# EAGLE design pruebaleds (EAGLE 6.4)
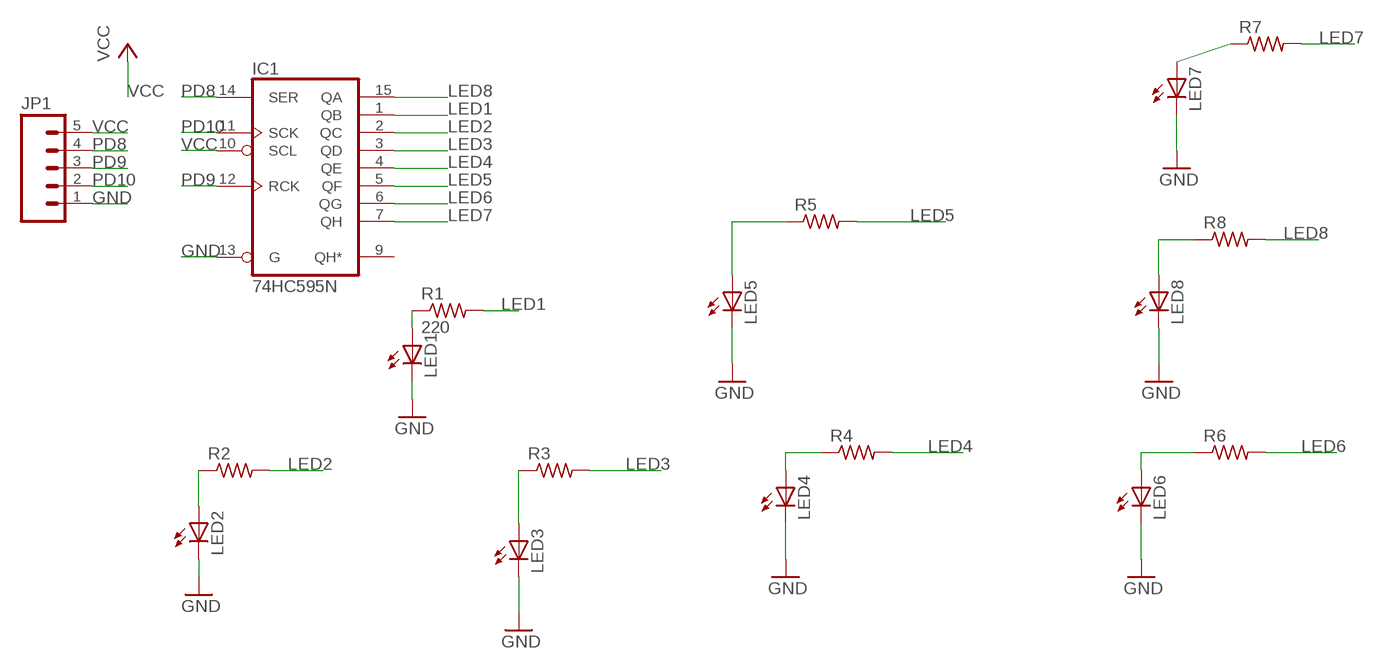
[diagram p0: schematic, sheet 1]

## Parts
IC1  74HC595N  [DIL16]
JP1  M05PTH  [1X05]
LED1  LED1206  [1206]
LED2  LED1206  [1206]
LED3  LED1206  [1206]
LED4  LED1206  [1206]
LED5  LED1206  [1206]
LED6  LED1206  [1206]
LED7  LED1206  [1206]
LED8  LED1206  [1206]
R1  220  RESISTOR1206  [1206]
R2  RESISTOR1206  [1206]
R3  RESISTOR1206  [1206]
R4  RESISTOR1206  [1206]
R5  RESISTOR1206  [1206]
R6  RESISTOR1206  [1206]
R7  RESISTOR1206  [1206]
R8  RESISTOR1206  [1206]

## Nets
GND: IC1.13(G) JP1.1 LED1.2(C) LED2.2(C) LED3.2(C) LED4.2(C) LED5.2(C) LED6.2(C) LED7.2(C) LED8.2(C)
LED1: IC1.1(QB) R1.2
LED2: IC1.2(QC) R2.2
LED3: IC1.3(QD) R3.2
LED4: IC1.4(QE) R4.2
LED5: IC1.5(QF) R5.2
LED6: IC1.6(QG) R6.2
LED7: IC1.7(QH) R7.2
LED8: IC1.15(QA) R8.2
N$1: LED2.1(A) R2.1
N$2: LED3.1(A) R3.1
N$3: LED4.1(A) R4.1
N$4: LED6.1(A) R6.1
N$5: LED8.1(A) R8.1
N$6: LED5.1(A) R5.1
N$7: LED7.1(A) R7.1
N$8: LED1.1(A) R1.1
PD8: IC1.14(SER) JP1.4
PD9: IC1.12(RCK) JP1.3
PD10: IC1.11(SCK) JP1.2
VCC: IC1.10(SCL) JP1.5
Unconnected: IC1.9(QH*)

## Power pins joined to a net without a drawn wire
GND: IC1.8(GND)
VCC: IC1.16(VCC)

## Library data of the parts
IC1 = 74xx-eu:74*595: 8-bit SHIFT REGISTER, output latch
JP1 = 01_SparkFun:M05: Header 5 Standard 5-pin 0.1" header. Use with straight break away headers (SKU : PRT-00116), right angle break away headers (PRT-00553), swiss pins (PRT-00743), machine pins (PRT-00117), and female headers (PRT-00115). Molex polarized connector foot print use with SKU : PRT-08230 with associated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
LED1-LED8 = 01_FAB_Hello:LED
R1-R8 = 01_FAB_Hello:RESISTOR

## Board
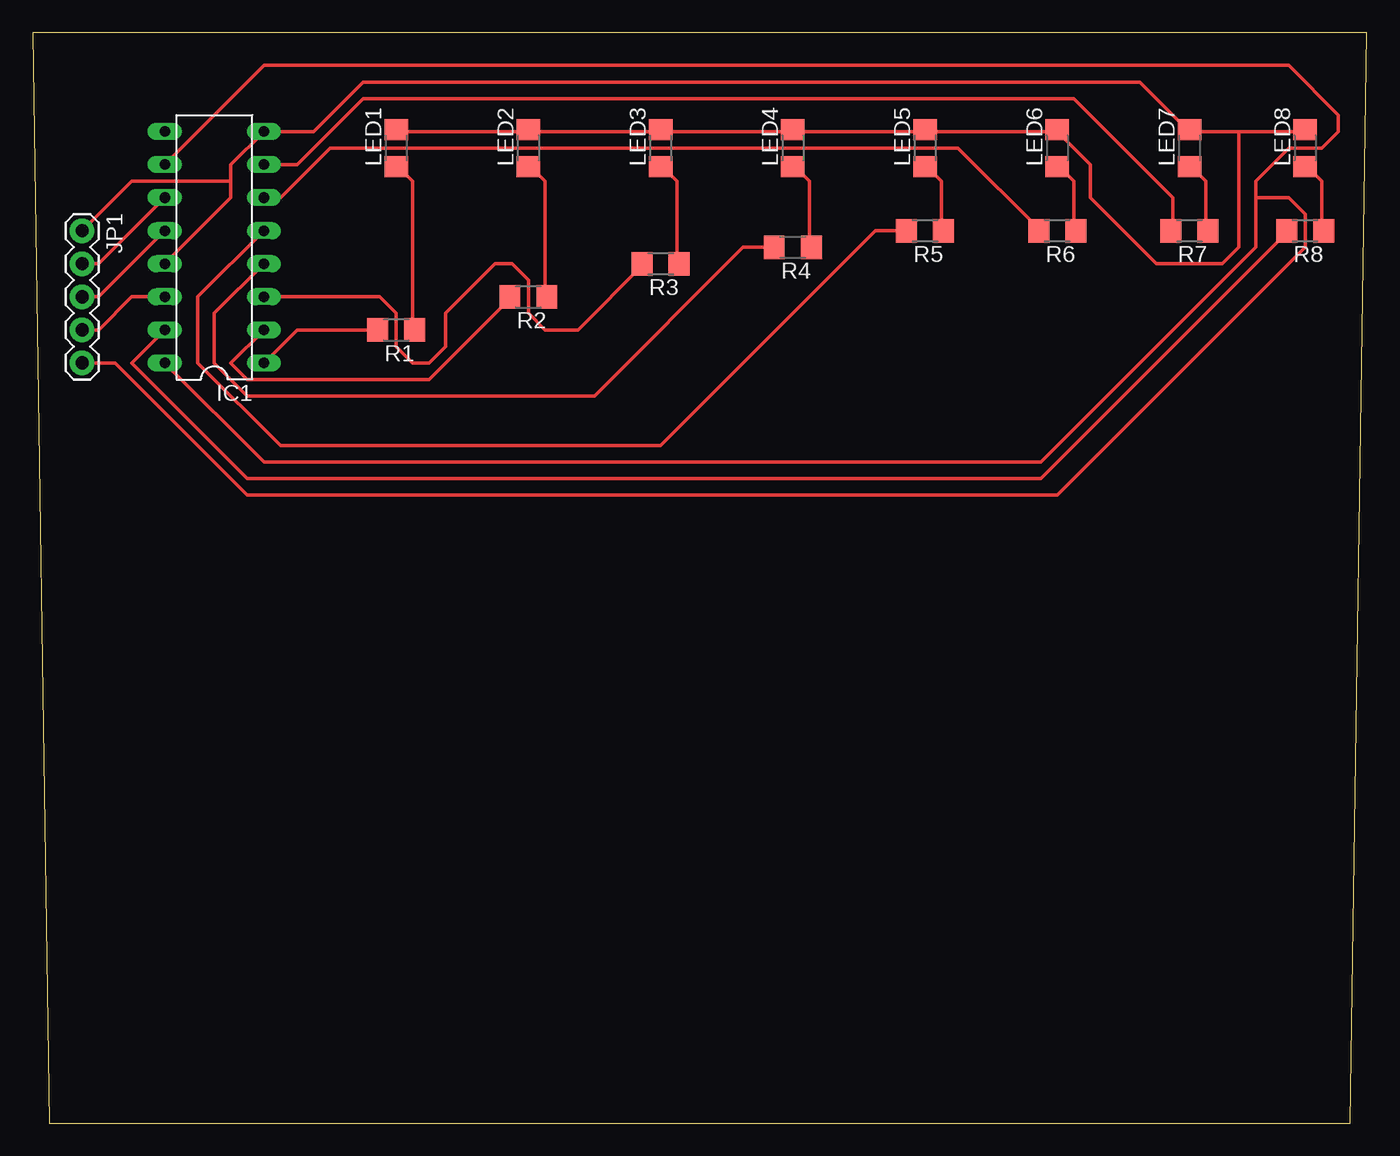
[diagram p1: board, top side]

Size 102.54 x 83.81 mm. Coordinates in mm from the lower left corner, seen from the top.
Outline: 1.27,0 101.27,0 102.54,83.81 0,83.81 1.27,0
Copper layers (1*16): Top 0.035mm / dielectric 1.5mm / Bottom 0.035mm
Design rules "default *": minimum track width 10mil, minimum drill 24mil, track to track 16mil, track to pad 16mil, pad to pad 16mil, via to via 16mil, smd to smd 0mil, copper to edge 40mil, drill to drill 8mil, minimum pad ring 10mil, minimum via ring 8mil, stop-mask expansion 4mil, vias tented up to drill 0mil, thermal gap 10mil

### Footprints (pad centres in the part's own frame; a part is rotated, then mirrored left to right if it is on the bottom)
DIL16 = drill 0.813 long: 1 -8.89,-3.81; 2 -6.35,-3.81; 3 -3.81,-3.81; 4 -1.27,-3.81; 5 1.27,-3.81; 6 3.81,-3.81; 7 6.35,-3.81; 8 8.89,-3.81; 9 8.89,3.81; 10 6.35,3.81; 11 3.81,3.81; 12 1.27,3.81; 13 -1.27,3.81; 14 -3.81,3.81; 15 -6.35,3.81; 16 -8.89,3.81
1X05 = drill 1.016 pad 1.88: 1 0,0; 2 2.54,0; 3 5.08,0; 4 7.62,0; 5 10.16,0
1206 = smd 1.6 x 1.803: 1 -1.422,0; 2 1.422,0

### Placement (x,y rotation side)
IC1  13.97,67.31 90 top
JP1  3.81,68.58 270 top
LED1  27.94,74.93 90 top
LED2  38.1,74.93 90 top
LED3  48.26,74.93 90 top
LED4  58.42,74.93 90 top
LED5  68.58,74.93 90 top
LED6  78.74,74.93 90 top
LED7  88.9,74.93 90 top
LED8  97.79,74.93 90 top
R1  27.94,60.96 180 top
R2  38.1,63.5 180 top
R3  48.26,66.04 180 top
R4  58.42,67.31 180 top
R5  68.58,68.58 180 top
R6  78.74,68.58 180 top
R7  88.9,68.58 180 top
R8  97.79,68.58 180 top

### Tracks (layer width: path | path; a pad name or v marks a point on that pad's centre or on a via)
GND
  Top 0.254: IC1.13 15.24,71.12 15.24,72.39 | 15.24,72.39 15.24,73.66 IC1.8 21.59,76.2 25.4,80.01 85.09,80.01 88.9,76.2 | JP1.1 7.62,72.39 15.24,72.39 | 92.71,76.2 97.79,76.2 LED8.2 | 92.71,76.2 88.9,76.2 | 38.1,76.2 27.94,76.2 LED1.2 | 38.1,76.2 48.26,76.2 | 38.1,76.2 LED2.2 | 48.26,76.2 58.42,76.2 | 48.26,76.2 LED3.2 | 58.42,76.2 68.58,76.2 | 58.42,76.2 LED4.2 | 68.58,76.2 78.74,76.2 | 68.58,76.2 LED5.2 | 92.71,76.2 92.71,67.31 91.44,66.04 86.36,66.04 81.28,71.12 81.28,73.66 78.74,76.2 | 78.74,76.2 LED6.2 | 88.9,76.2 LED7.2
LED1
  Top 0.254: IC1.1 20.32,60.96 R1.2 26.67,60.96
LED2
  Top 0.254: IC1.2 15.24,58.42 16.51,57.15 30.48,57.15 36.83,63.5 R2.2
LED3
  Top 0.254: IC1.3 26.67,63.5 27.94,62.23 27.94,59.69 29.21,58.42 30.48,58.42 31.75,59.69 31.75,62.23 35.56,66.04 36.83,66.04 38.1,64.77 38.1,62.23 39.37,60.96 41.91,60.96 46.99,66.04 R3.2
LED4
  Top 0.254: IC1.4 13.97,62.23 13.97,58.42 16.51,55.88 43.18,55.88 54.61,67.31 R4.2 57.15,67.31
LED5
  Top 0.254: IC1.5 12.7,63.5 12.7,58.42 19.05,52.07 48.26,52.07 64.77,68.58 R5.2 67.31,68.58
LED6
  Top 0.254: IC1.6 19.05,71.12 22.86,74.93 71.12,74.93 77.47,68.58 R6.2
LED7
  Top 0.254: IC1.7 20.32,73.66 25.4,78.74 80.01,78.74 87.63,71.12 87.63,68.58 R7.2
LED8
  Top 0.254: IC1.15 7.62,58.42 16.51,49.53 77.47,49.53 96.52,68.58 R8.2
N$1
  Top 0.254: R2.1 39.37,63.5 39.37,72.39 38.1,73.66 LED2.1
N$2
  Top 0.254: R3.1 49.53,66.04 49.53,72.39 48.26,73.66 LED3.1
N$3
  Top 0.254: R4.1 59.69,67.31 59.69,72.39 58.42,73.66 LED4.1
N$4
  Top 0.254: R6.1 80.01,68.58 80.01,72.39 78.74,73.66 LED6.1
N$5
  Top 0.254: R8.1 99.06,68.58 99.06,72.39 97.79,73.66 LED8.1
N$6
  Top 0.254: R5.1 69.85,68.58 69.85,72.39 68.58,73.66 LED5.1
N$7
  Top 0.254: R7.1 90.17,68.58 90.17,72.39 88.9,73.66 LED7.1
N$8
  Top 0.254: R1.1 29.21,60.96 29.21,72.39 27.94,73.66 LED1.1
PD8
  Top 0.254: IC1.14 7.62,63.5 5.08,60.96 JP1.4
PD9
  Top 0.254: IC1.12 5.08,63.5 JP1.3
PD10
  Top 0.254: IC1.11 5.08,66.04 JP1.2
VCC
  Top 0.254: IC1.16 17.78,50.8 77.47,50.8 93.98,67.31 93.98,71.12 | 93.98,71.12 93.98,72.39 96.52,74.93 99.06,74.93 100.33,76.2 100.33,77.47 96.52,81.28 17.78,81.28 IC1.10 | JP1.5 6.35,58.42 16.51,48.26 78.74,48.26 97.79,67.31 97.79,69.85 96.52,71.12 93.98,71.12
